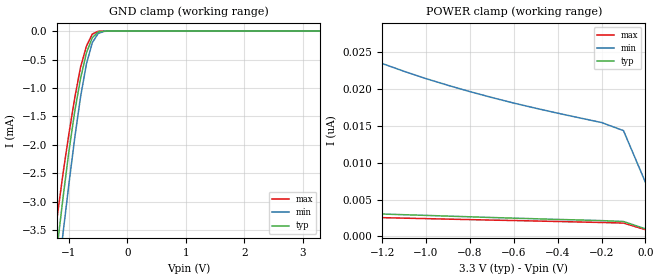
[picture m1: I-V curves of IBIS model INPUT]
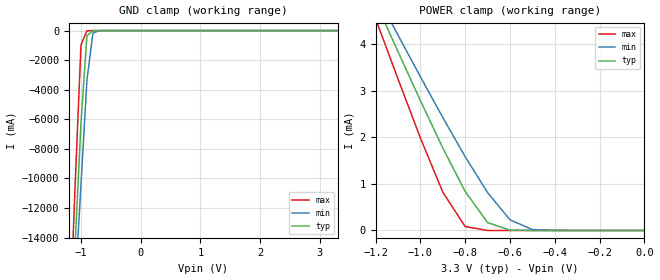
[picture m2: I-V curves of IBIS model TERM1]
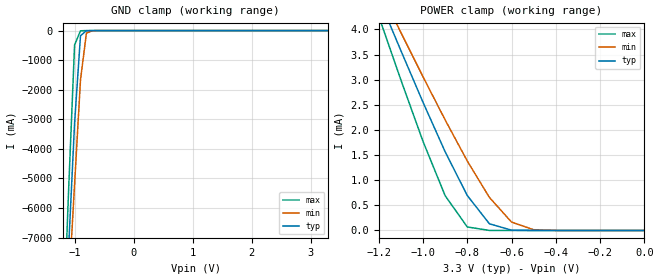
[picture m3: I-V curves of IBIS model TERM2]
|   DIODES INCORPORATED
|   IBIS Model of PI3B3251
|   Product Family: 3B
|   TSSOP (L) Package
[IBIS Ver] 3.2
[Comment char] |_char
[File Name] pi3b3251_l_33v.ibs
[File Rev] 1.0
[Source] File originated at Diodes Incorporated.
[Date] 10/15/15
[Disclaimer] (C) Copyright DIODES INCORPORATED
   All rights reserved
  Diodes Incorporated hereby grants the user of
  this IBIS model a non-exclusive, nontransferable license to
  use this IBIS model under the following terms.
  This IBIS model is provided on an "AS IS" basis and Diodes
  makes absolutely no warranty with respect to the information
  contained herein. DIODES DISCLAIMS AND CUSTOMER WAIVES ALL
  WARRANTIES, EXPRESSED OR IMPLIED, INCLUDING WARRANTIES OF
  MERCHANTABILITY OR FITNESS FOR A PARTICULAR PURPOSE. The
  entire risk as to quality and performance is with the customer.
  Accordingly, in no event shall the company be liable for any
  damages, whether in contract or tort, including any lost
  profits or other incidental, consequential, exemplary, or
  punitive damages arising out of the use or application of the
  IBIS model provided in this package. Further, Diodes reserves
  the right to make changes without notice to any product herein
  to improve reliability, function, or design. Diodes does not
  convey any license under patent rights or any other intellectual
  property rights, including those of third parties.
  The user is granted this license only to use the IBIS model
  and is not granted rights to sell, load, rent, lease or license
  the IBIS model in whole or in part, or in modified form to anyone
  other than user. User may modify the IBIS model to suit its specific
  application but rights to derivative works and such modifications
  shall belong to Diodes.
  Diodes is not obligated to provide maintenance or support
  for the licensed IBIS model.
  Contact Diodes at ATTN: APPLICATION ENGINEERING / IBIS MODELS
  1545 Barber Ln. Milpitas, CA 95035
[Component] PI3B3251
[Manufacturer] Diodes Incorporated.
[Package]
| variable   typ   min   max
R_pkg   0.05666ohm   0.05334ohm   0.05997ohm
L_pkg   2.99150nH   2.22200nH   3.76100nH
C_pkg   0.20800pF   0.16300pF   0.25300pF
[Pin]   signal_name  model_name  R_pin   L_pin   C_pin
1   I3   TERM1   0.05997   3.76100nH   0.25300pF
2   I2   TERM1   0.05776   3.24800nH   0.22300pF
3   I1   TERM1   0.05555   2.73500nH   0.19300pF
4   I0   TERM1   0.05334   2.22200nH   0.16300pF
5   Y   TERM2   0.05334   2.22200nH   0.16300pF
6   NC   NC   0.05555   2.73500nH   0.19300pF
7   _E   INPUT   0.05776   3.24800nH   0.22300pF
8   GND   GND   0.05997   3.76100nH   0.25300pF
9   S2   INPUT   0.05997   3.76100nH   0.25300pF
10   S1   INPUT   0.05776   3.24800nH   0.22300pF
11   S0   INPUT   0.05555   2.73500nH   0.19300pF
12   I7   TERM1   0.05334   2.22200nH   0.16300pF
13   I6   TERM1   0.05334   2.22200nH   0.16300pF
14   I5   TERM1   0.05555   2.73500nH   0.19300pF
15   I4   TERM1   0.05776   3.24800nH   0.22300pF
16   VCC   POWER   0.05997   3.76100nH   0.25300pF
[Series Switch Groups]
On 1 /
Off 2 3 4 5 6 7 8 /
[Series Pin Mapping]   pin_2   model_name  function_table_group
1   5   SWITCH1   1
2   5   SWITCH1   2
3   5   SWITCH1   3
4   5   SWITCH1   4
15   5   SWITCH1   5
14   5   SWITCH1   6
13   5   SWITCH1   7
12   5   SWITCH1   8
|   Model SWITCH1
[Model] SWITCH1
Model_type Series_switch
| variable   typ   min   max
C_comp   10.500pF   10.200pF   10.800pF
[Voltage Range]   3.3000V   2.9700V   3.6300V
[GND Clamp Reference]   0.0000V   0.0000V   0.0000V
[POWER Clamp Reference]   3.3000V   2.9700V   3.6300V
[Temperature Range]   25   85   -40
[On]
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[OFF]
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| Models and submodels in the file (4): INPUT (Input), SWITCH1 (Series_switch), TERM1 (Terminator), TERM2 (Terminator)
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|   Model INPUT
[Model] INPUT
Model_type Input
Vinl = 800mV
Vinh = 2.0V
| variable   typ   min   max
C_comp   3.000pF   2.900pF   3.100pF
[Voltage Range]   3.3000V   2.9700V   3.6300V
[GND Clamp Reference]   0.0000V   0.0000V   0.0000V
[POWER Clamp Reference]   3.3000V   2.9700V   3.6300V
[Temperature Range]   25   85   -40
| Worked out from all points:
|   GND clamp passes 1 mA (typ) near -0.83 V on its own axis
[GND Clamp]
| Voltage   I(typ)   I(min)   I(max)
-3.3V     -24.17mA   -24.42mA   -24.09mA
-1.3V     -4.71mA    -5.353mA   -4.125mA
-1.2V     -3.802mA   -4.445mA   -3.269mA
-1.1V     -2.929mA   -3.554mA   -2.501mA
-1V       -2.118mA   -2.692mA   -1.809mA
-900mV    -1.411mA   -1.878mA   -1.173mA
-800mV    -829.8uA   -1.151mA   -632.5uA
-700mV    -381.7uA   -576.7uA   -263uA
-600mV    -116.2uA   -203.6uA   -52.63uA
-500mV    -16.3uA    -42uA      -3.416uA
-400mV    -1.145uA   -5.033uA   -91.97nA
3.3V      1.01nA     16.27nA    23.98pA
[POWER Clamp]   |Note: Vtable = Vcc - Voutput
| Voltage   I(typ)   I(min)   I(max)
-3.3V     6.818nA    89.17nA    3.932nA
-3V       5.933nA    71.31nA    3.74nA
-2.5V     4.813nA    49.93nA    3.389nA
-1.6V     3.476nA    28.72nA    2.808nA
-1.5V     3.356nA    27.24nA    2.739nA
-1.3V     3.13nA     24.63nA    2.602nA
-1V       2.842nA    21.42nA    2.402nA
-800mV    2.65nA     19.66nA    2.268nA
-600mV    2.465nA    18.1nA     2.143nA
-200mV    2.132nA    15.46nA    1.877nA
-100mV    2.012nA    14.35nA    1.799nA
0V        1.01nA     7.337nA    893.5pA
|   Model TERM1
[Model] TERM1
Model_type Terminator
| variable   typ   min   max
C_comp   7.000pF   6.800pF   7.200pF
[Voltage Range]   3.3000V   2.9700V   3.6300V
[GND Clamp Reference]   0.0000V   0.0000V   0.0000V
[POWER Clamp Reference]   3.3000V   2.9700V   3.6300V
[Temperature Range]   25   85   -40
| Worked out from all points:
|   GND clamp passes 1 mA (typ) near -0.71 V on its own axis
|   POWER clamp passes 1 mA (typ) near -0.82 V on its own axis
[GND Clamp]
| Voltage   I(typ)   I(min)   I(max)
-3.3V     -198.2A    -172.9A    -239.3A
-1.2V     -22.95A    -24.52A    -21.07A
-1.1V     -14.6A     -17.46A    -10.67A
-1V       -6.255A    -10.4A     -968.6mA
-900mV    -345.5mA   -3.339A    -11.3mA
-800mV    -10.61mA   -172.3mA   -151.5uA
-700mV    -350.4uA   -9.392mA   -1.276uA
3.3V      786.5pA    112.3nA    110.4pA
[POWER Clamp]   |Note: Vtable = Vcc - Voutput
| Voltage   I(typ)   I(min)   I(max)
-3.3V     26.63mA    24.59mA    29.73mA
-1.2V     4.898mA    5.094mA    4.542mA
-1.1V     3.836mA    4.191mA    3.25mA
-1V       2.787mA    3.298mA    1.985mA
-900mV    1.77mA     2.423mA    821.9uA
-800mV    836.8uA    1.582mA    82.7uA
-700mV    169.7uA    811.8uA    826.1nA
-600mV    6.664uA    229.3uA    8.305nA
-500mV    147.7nA    20.06uA    2.399nA
-400mV    5.577nA    918.8nA    2.265nA
0V        786.5pA    4.94nA     722pA
|   Model TERM2
[Model] TERM2
Model_type Terminator
| variable   typ   min   max
C_comp   3.500pF   3.4000pF   3.600pF
[Voltage Range]   3.3000V   2.9700V   3.6300V
[GND Clamp Reference]   0.0000V   0.0000V   0.0000V
[POWER Clamp Reference]   3.3000V   2.9700V   3.6300V
[Temperature Range]   25   85   -40
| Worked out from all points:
|   GND clamp passes 1 mA (typ) near -0.71 V on its own axis
|   POWER clamp passes 1 mA (typ) near -0.83 V on its own axis
[GND Clamp]
| Voltage   I(typ)   I(min)   I(max)
-3.3V     -99.12A    -86.44A    -119.7A
-1.2V     -11.47A    -12.26A    -10.53A
-1.1V     -7.301A    -8.73A     -5.338A
-1V       -3.129A    -5.2A      -486.2mA
-900mV    -174.2mA   -1.671A    -6.956mA
-800mV    -6.311mA   -87.22mA   -146.7uA
-700mV    -315.8uA   -5.394mA   -1.275uA
3.3V      730.4pA    102.9nA    65.03pA
[POWER Clamp]   |Note: Vtable = Vcc - Voutput
| Voltage   I(typ)   I(min)   I(max)
-3.3V     26.24mA    24.2mA     29.33mA
-1.2V     4.628mA    4.834mA    4.266mA
-1.1V     3.58mA     3.941mA    2.998mA
-1V       2.552mA    3.06mA     1.774mA
-900mV    1.567mA    2.201mA    692.7uA
-800mV    695.9uA    1.383mA    70.32uA
-700mV    133.2uA    657.6uA    811.8nA
-600mV    6.007uA    166.8uA    8.287nA
-500mV    143.5nA    15.36uA    2.397nA
0V        730.8pA    4.881nA    663pA
